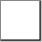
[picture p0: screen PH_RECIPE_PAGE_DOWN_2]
VISUALIZATION PH_RECIPE_PAGE_DOWN_2  // 42x42
VAR_IN_OUT
	RECIPE_CTRL_V2 : None;
END_VAR
    Rectangle (0,0 40x40)
        tap RECIPE_CTRL_V2.sCmd.bPageDown
    Polygon (20,20), colour toggle: (RECIPE_CTRL_V2.sCmd.bPageDown) <> 0
        tap RECIPE_CTRL_V2.sCmd.bPageDown
    Polygon (20,30), colour toggle: (RECIPE_CTRL_V2.sCmd.bPageDown) <> 0
        tap RECIPE_CTRL_V2.sCmd.bPageDown
END_VISUALIZATION
